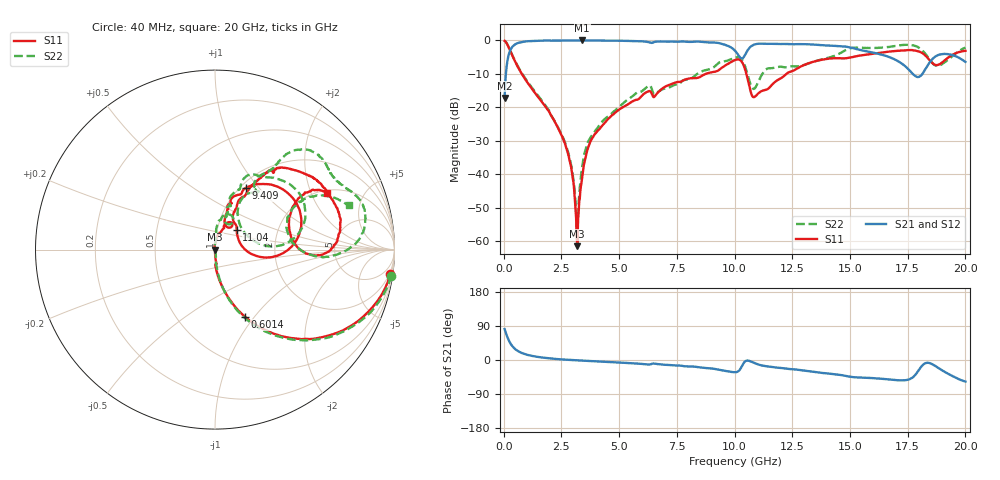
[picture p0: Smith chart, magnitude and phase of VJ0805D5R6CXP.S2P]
! VJ0805D5R6CXP
! DATE 10/29/2021  11:54
! CAPACITORS MOUNTED IN SERIES ON 25 MIL THICK MICROSTRIP SUBSTRATE
# GHz  S  MA  R  50.00
!  FREQ  S11M  S11A  S21M  S21A  S12M  S12A  S22M  S22A
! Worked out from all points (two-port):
!   1601 points, 40 MHz to 20 GHz, reference 50 ohm
!   highest |S21| = 0.01 dB at 3.396 GHz (marker M1); lowest = -17.2 dB at 40 MHz (marker M2)
!   |S21| within 3 dB of the highest: 282.1 MHz to 10.01 GHz (9.729 GHz wide, 189 % of centre); 10.56 GHz to 15.55 GHz (4.985 GHz wide, 38.2 % of centre)
!   lowest |S11| = -61.5 dB at 3.184 GHz (marker M3), VSWR 1.00, Z = 50.1 + j0.015 ohm
!   |S11| at or under -10 dB: 786.1 MHz to 8.746 GHz (7.96 GHz wide, 167 % of centre); 10.51 GHz to 12.24 GHz (1.728 GHz wide, 15.2 % of centre)
!   |S22| runs from -59.2 to -0.1 dB; largest |S21 - S12| = 0.0067
!   S11 on the Smith chart (normalised r, x): 40 MHz: 1, -14; 601.4 MHz: 1.00, -0.90; 9.409 GHz: 1.06, +0.85; 11.04 GHz: 1.24, +0.28; 20 GHz: 2.14, +2.62
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0.04  0.9858 -8.1  0.1388 81.4  0.1401 81.1  0.9927 -8.4
0.2396  0.758 -40.4  0.6481 49.4  0.6479 49.5  0.7662 -40.6
0.601375  0.4094 -66.0  0.9119 24.3  0.9118 24.1  0.4184 -66.3
2.5849  0.03321 -88.2  0.9968 1.3  0.9966 1.2  0.03443 -82.6
2.921725  0.013 -88.8  0.9978 0.1  0.9979 -0.1  0.01375 -78.3
3.1837  0.0008434 10.2  0.9987 -0.8  0.9994 -0.9  0.0011 16.6
3.370825  0.007506 92.3  1 -1.4  1 -1.5  0.01073 100.0
3.395775  0.008712 93.5  1.001 -1.6  1.001 -1.6  0.01259 100.2
3.720125  0.02867 92.3  0.9984 -2.5  0.9989 -2.7  0.03353 88.3
4.368825  0.058 83.4  0.9948 -4.4  0.9954 -4.5  0.06692 84.9
6.70165  0.1699 71.6  0.9652 -11.0  0.9653 -11.1  0.1721 71.7
9.408725  0.383 63.7  0.8971 -26.9  0.8976 -27.0  0.4751 60.7
10.02  0.5101 39.3  0.7037 -32.2  0.7039 -32.5  0.553 41.4
10.53148  0.3 -8.4  0.6805 -1.7  0.6816 -1.8  0.3395 3.1
11.04295  0.1634 42.2  0.8944 -12.1  0.8953 -12.2  0.2465 59.2
13.35083  0.4739 57.4  0.8707 -30.8  0.87 -31.0  0.4711 59.1
14.9102  0.5467 53.0  0.7998 -43.0  0.8004 -43.4  0.7434 48.7
16.68165  0.6821 35.5  0.5678 -51.3  0.5681 -51.6  0.7997 26.0
17.72955  0.7125 12.0  0.3143 -45.3  0.3152 -45.6  0.8472 9.2
18.31587  0.5755 -3.0  0.3991 -7.5  0.3981 -7.8  0.6002 -4.1
18.93962  0.4541 23.8  0.622 -25.4  0.6237 -25.7  0.4329 21.7
20  0.6994 26.7  0.4783 -56.9  0.4783 -57.3  0.7851 18.4
